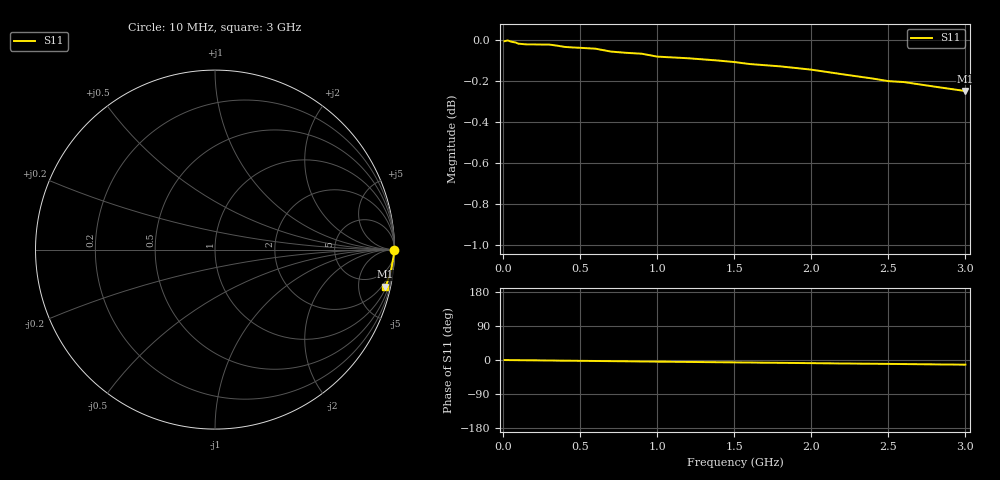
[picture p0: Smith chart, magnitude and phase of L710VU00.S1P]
! SIEMENS Small Signal Semiconductors
! BAR14-1
! Si PIN Diode in SOT23
! VR = 10 V
! S-Parameters:  July  1992
# GHz  S  MA  R  50
!  f  S11
! GHz  MAG  ANG
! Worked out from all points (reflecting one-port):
!   31 points, 10 MHz to 3 GHz, reference 50 ohm
!   lowest |S11| = -0.2 dB at 3 GHz (marker M1), VSWR 69.67, Z = 61.4 - j456 ohm
!   phase of S11 starts at -0 deg and turns -12 deg over the sweep
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0.01  0.9992 -0.1
0.03  0.9996 -0.2
0.05  0.999 -0.3
0.06  0.9988 -0.3
0.08  0.9985 -0.4
0.1  0.9978 -0.5
0.15  0.9974 -0.7
0.2  0.9974 -0.9
0.3  0.9973 -1.3
0.35  0.9967 -1.6
0.4  0.996 -1.8
0.6  0.995 -2.6
0.7  0.9934 -3.0
0.8  0.9927 -3.4
0.9  0.9922 -3.9
1  0.9906 -4.3
1.2  0.9897 -5.1
1.4  0.9884 -5.9
1.5  0.9876 -6.3
1.6  0.9865 -6.7
1.8  0.9852 -7.5
2  0.9834 -8.3
2.2  0.9809 -9.2
2.4  0.9785 -9.9
2.5  0.9771 -10.3
2.6  0.9766 -10.7
2.8  0.9741 -11.6
3  0.9717 -12.3
